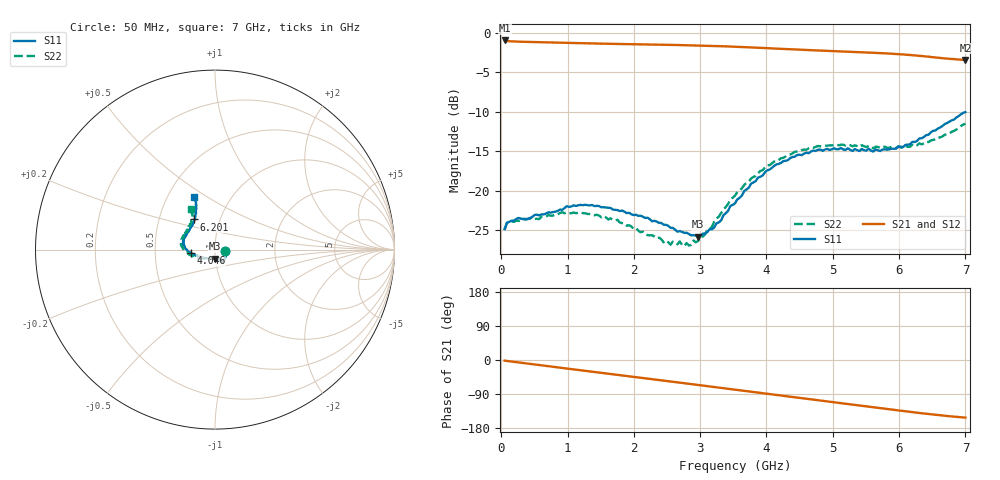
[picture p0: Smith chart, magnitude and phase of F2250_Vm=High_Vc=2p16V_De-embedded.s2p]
! Integrated Device Technology
! Corporate Headquarters
! 6024 Silver Creek Valley Road
! San Jose, CA 95138  USA
! Phone:  1-408-284-8200
! Toll Free:  1-800-223-1366
! Webpage:  http://www.idt.com/
! Timing and RF Division
! 515 Groton Road, Suite 102
! Westford, MA 01886-6024
! Device:  F2250
! Description: Voltage Variable RF Attenuator
! Frequency:  50.0 -  6000.00 MHz
! Package:  3x3 mm Thin QFN Plastic Package: 16 pin
! Ports:  2 RF, 3 DC
!  Pin  1  = GND
!  Pin  2  = NC
!  Pin  3  = RF1  = Port 1
!  Pin  4  = NC
!  Pin  5  = GND
!  Pin  6  = GND
!  Pin  7  = GND
!  Pin  8  = GND
!  Pin  9  = NC
!  Pin 10  = RF2  = Port 2
!  Pin 11  = NC
!  Pin 12  = GND
!  Pin 13  = GND
!  Pin 14  = VCNTRL
!  Pin 15  = VDD
!  Pin 16  = VMODE
! Vcntrl:  2.160 Volts
! Vmode:  +3.300 Volts
! Vdd:  +3.30  Volts
! Current:  1.318 mA
! Data:  The device was measured on a the F2250 evaluation board which has
!  individual transmission lines to the RF pins.  Data was collected
!  using a calibrated network analyzer.  The evaluation board was
!  de-embedded using a TRL calibration technique.
!  The reference plane is the edge of the package pin.
! Misc:  SN 10
!  Action Tracker AT0258
! Date Measured:  2014-11-26
! Date:  2015-10-15  MJV
! Note:
!  Integrated Device Technology supplies this data as a sample of measured
!  data at the package pin for this product.  Your particular data for this
!  product may vary.
!  Data was taken at 25 degrees C.
!  Integrated Device Technology reserves the right to change this data at anytime.
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# GHz S dB R 50
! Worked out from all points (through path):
!   201 points, 50 MHz to 7 GHz, reference 50 ohm
!   highest |S21| = -0.94 dB at 50 MHz (marker M1); lowest = -3.4 dB at 7 GHz (marker M2)
!   group delay of S21, straight-line fit = 61.1 ps
!   lowest |S11| = -25.8 dB at 2.969 GHz (marker M3), VSWR 1.11, Z = 49.5 - j5.07 ohm
!   |S11| at or under -10 dB: start of sweep to end of sweep
!   |S22| runs from -27.0 to -11.5 dB; largest |S21 - S12| = 0.0019
!   S11 on the Smith chart (normalised r, x): 50 MHz: 1.12, -0.02; 4.046 GHz: 0.76, -0.03; 6.201 GHz: 0.75, +0.26; 7 GHz: 0.68, +0.44
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0.05  -24.83 -9.7  -0.94 -1.8  -0.94 -1.8  -25.02 -10.2
0.1195  -23.94 -9.5  -1.04 -3.2  -1.04 -3.2  -23.91 -8.5
0.57125  -23.12 -29.5  -1.16 -13.3  -1.16 -13.3  -23.60 -30.4
0.91875  -22.42 -47.5  -1.23 -21.0  -1.23 -21.1  -22.72 -49.5
1.2315  -21.83 -55.3  -1.29 -27.9  -1.29 -27.9  -22.84 -59.9
1.75275  -22.45 -62.2  -1.39 -39.1  -1.39 -39.1  -23.69 -66.9
2.37825  -24.09 -62.3  -1.48 -52.8  -1.48 -52.8  -25.95 -68.1
2.552  -24.70 -66.8  -1.50 -56.6  -1.50 -56.7  -26.84 -74.7
2.691  -25.12 -74.2  -1.53 -59.7  -1.53 -59.8  -26.43 -82.0
2.7605  -25.35 -76.3  -1.54 -61.3  -1.54 -61.3  -27.03 -86.3
2.969  -25.83 -92.9  -1.58 -66.0  -1.58 -66.0  -26.37 -104.6
3.21225  -24.66 -122.6  -1.63 -71.4  -1.63 -71.5  -23.90 -128.9
3.525  -21.60 -148.9  -1.73 -78.5  -1.73 -78.5  -20.62 -147.5
3.76825  -19.09 -162.0  -1.82 -84.0  -1.82 -84.0  -18.45 -158.7
4.04625  -17.31 -171.8  -1.94 -90.2  -1.93 -90.2  -16.76 -169.2
4.4285  -15.68 177.7  -2.08 -98.6  -2.08 -98.6  -15.06 179.3
4.7065  -14.90 170.7  -2.18 -104.8  -2.18 -104.8  -14.55 173.5
5.054  -14.75 162.4  -2.31 -112.4  -2.31 -112.5  -14.16 166.4
5.85325  -14.75 136.4  -2.61 -130.0  -2.61 -130.1  -14.57 147.5
6.20075  -13.80 124.6  -2.82 -137.7  -2.82 -137.8  -14.16 138.5
6.54825  -12.35 116.4  -3.09 -144.7  -3.09 -144.8  -13.51 127.1
7  -10.03 111.4  -3.42 -152.1  -3.43 -152.2  -11.49 120.8
